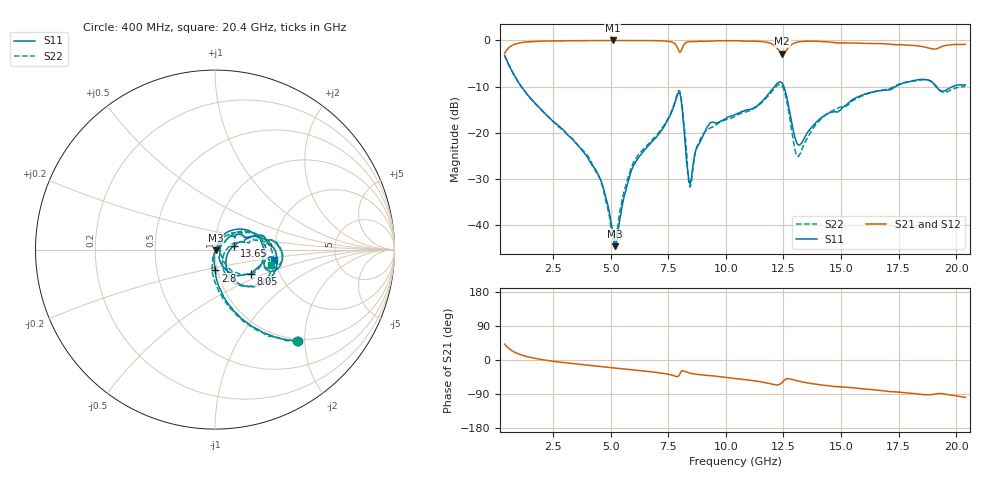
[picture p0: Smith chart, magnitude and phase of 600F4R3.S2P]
!  American Technical Ceramics  Date:  11/23/05
!  One Norden Lane
!  Huntington Station,  NY.  11746-2102
!  Tel:  (631) 622-4700  Fax:  (631) 622-4748
!  Part Number  600F4R3  Mounting Orientation: Horizontal
!  Description: Ultra Low ESR Microwave capacitors
!  Application: Coupling, Bypass, Tuning, DC Block
!  Filters, Matching
# GHZ S DB R 50
! Freq  |S11|  S11 Ph  |S21|  S21 Ph  |S12|  S12 Ph  |S22|  S22 Ph
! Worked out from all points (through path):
!   401 points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, 400 MHz to 20.4 GHz, reference 50 ohm
!   highest |S21| = 0.00 dB at 5.1 GHz (marker M1); lowest = -2.9 dB at 12.45 GHz (marker M2)
!   group delay of S21, straight-line fit = 15.2 ps
!   lowest |S11| = -44.5 dB at 5.2 GHz (marker M3), VSWR 1.01, Z = 50.5 - j0.298 ohm
!   |S11| at or under -10 dB: 1.13 GHz to 12.11 GHz (10.98 GHz wide, 166 % of centre); 12.52 GHz to 17.36 GHz (4.84 GHz wide, 32.4 % of centre); 19.15 GHz to 19.83 GHz (681 MHz wide, 3.49 % of centre)
!   |S22| runs from -44.3 to -3.3 dB; largest |S21 - S12| = 0.0065
!   S11 on the Smith chart (normalised r, x): 400 MHz: 0.97, -1.86; 2.8 GHz: 0.98, -0.23; 8.05 GHz: 1.43, -0.41; 13.65 GHz: 1.24, +0.05; 20.4 GHz: 1.95, -0.25
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0.4  -3.26 -47.7  -2.83 41.7  -2.84 41.6  -3.26 -48.1
1.15  -10.13 -76.1  -0.45 12.9  -0.45 13.0  -10.12 -77.6
2.8  -18.69 -89.3  -0.10 -5.7  -0.10 -5.6  -18.85 -98.1
3.75  -23.65 -94.1  -0.03 -12.2  -0.04 -12.2  -23.50 -101.6
4.6  -30.61 -99.8  -0.02 -17.5  -0.02 -17.5  -30.71 -102.4
5.1  -41.63 -62.1  0.00 -20.6  -0.01 -20.6  -43.05 -56.6
5.2  -44.47 -29.6  -0.01 -21.2  -0.01 -21.2  -44.30 -15.1
5.95  -27.54 63.2  0.00 -26.1  -0.01 -26.0  -26.92 44.2
7.1  -20.20 59.4  -0.06 -33.7  -0.05 -33.7  -19.84 41.7
7.75  -14.16 35.1  -0.55 -41.5  -0.56 -41.5  -13.88 30.8
8.05  -12.40 -34.2  -2.37 -31.6  -2.34 -31.7  -11.88 -30.6
8.35  -28.29 -45.2  -0.31 -33.0  -0.31 -33.0  -28.31 -38.8
8.45  -31.04 -2.2  -0.24 -34.8  -0.24 -34.8  -31.72 6.5
9.05  -20.19 42.2  -0.19 -39.9  -0.19 -39.9  -20.00 50.6
10.4  -16.04 33.2  -0.05 -49.1  -0.07 -49.0  -16.45 39.6
11.9  -11.34 13.6  -0.56 -62.1  -0.55 -62.1  -11.63 17.0
12.45  -9.20 -29.5  -2.89 -59.0  -2.88 -58.9  -9.92 -33.2
13.1  -22.33 -33.0  -0.37 -54.8  -0.38 -54.8  -24.99 -29.5
13.65  -19.19 11.3  -0.15 -61.3  -0.17 -61.3  -20.13 17.5
13.75  -18.64 13.0  -0.16 -62.3  -0.16 -62.3  -19.28 18.9
17.1  -10.68 10.1  -0.80 -83.2  -0.77 -83.1  -10.42 9.1
20.4  -9.59 -9.8  -0.86 -98.7  -0.85 -98.6  -9.88 -15.3
